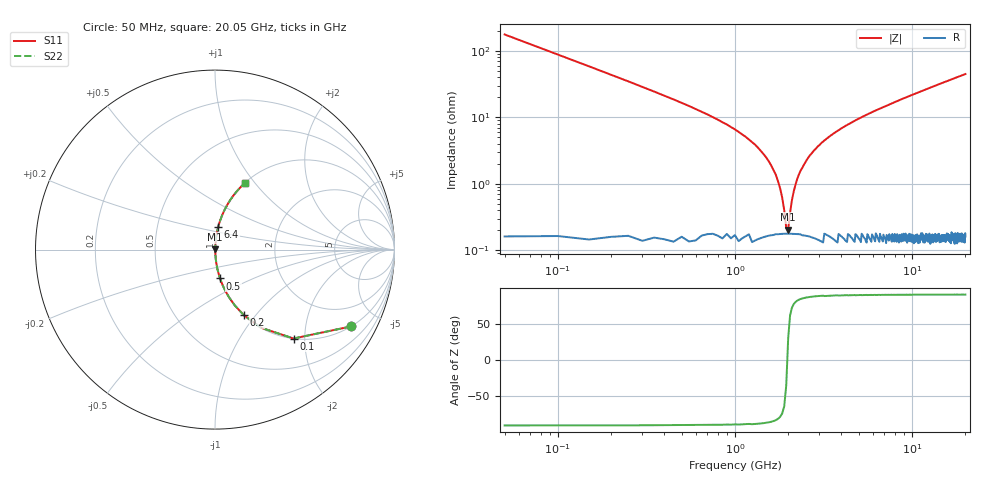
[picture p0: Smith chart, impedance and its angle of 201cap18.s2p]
! AVX Thin Film Operation		Date: May 2007
! Description: Accu-P® Series, Thin Film, SMD, RF Capacitor
! Part Number: 0201ZK180FBS
! 50 MHz  -  20.05 GHz
! Serial Measurements
# MHZ S MA R 50
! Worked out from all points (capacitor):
!   401 points, 50 MHz to 20.05 GHz, reference 50 ohm
!   read as one part in series: C = 18 pF near 150 MHz
!   lowest |Z| = 205 mohm at 2 GHz (marker M1)
!   series resonance near 1.977 GHz, so ESL is about 360 pH
!   S11 on the Smith chart (normalised r, x): 50 MHz: 1.00, -3.53; 100 MHz: 1.00, -1.76; 200 MHz: 1.00, -0.87; 500 MHz: 1.00, -0.33; 6.4 GHz: 1.00, +0.26; 20.05 GHz: 1.00, +0.90
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50  0.87 -29.5  0.492 60.5  0.492 60.5  0.87 -29.5
100  0.661 -48.5  0.749 41.4  0.749 41.4  0.661 -48.5
200  0.4 -66.2  0.915 23.6  0.915 23.6  0.4 -66.2
300  0.276 -73.7  0.96 16.0  0.96 16.0  0.276 -73.7
500  0.163 -80.1  0.985 9.4  0.985 9.4  0.163 -80.1
1250  0.042 -85.5  0.998 2.4  0.998 2.4  0.042 -85.5
1550  0.022 -84.7  0.998 1.3  0.998 1.3  0.022 -84.7
1750  0.011 -81.3  0.998 0.6  0.998 0.6  0.011 -81.3
1900  0.003876 -66.3  0.998 0.2  0.998 0.2  0.003876 -66.3
2000  0.001858 33.5  0.998 -0.1  0.998 -0.1  0.001858 33.5
2050  0.003585 64.2  0.998 -0.2  0.998 -0.2  0.003585 64.2
2200  0.009681 80.3  0.998 -0.5  0.998 -0.5  0.009681 80.3
2400  0.017 83.9  0.998 -1.0  0.998 -1.0  0.017 83.9
2750  0.03 85.3  0.998 -1.7  0.998 -1.7  0.03 85.3
3400  0.051 85.3  0.997 -2.9  0.997 -2.9  0.051 85.3
4600  0.084 84.1  0.995 -4.8  0.995 -4.8  0.084 84.1
6400  0.13 81.9  0.99 -7.4  0.99 -7.4  0.13 81.9
6750  0.138 81.4  0.989 -7.9  0.989 -7.9  0.138 81.4
10050  0.213 77.3  0.976 -12.3  0.976 -12.3  0.213 77.3
13400  0.284 73.2  0.957 -16.5  0.957 -16.5  0.284 73.2
16750  0.349 69.3  0.935 -20.5  0.935 -20.5  0.349 69.3
20050  0.409 65.7  0.911 -24.2  0.911 -24.2  0.409 65.7
